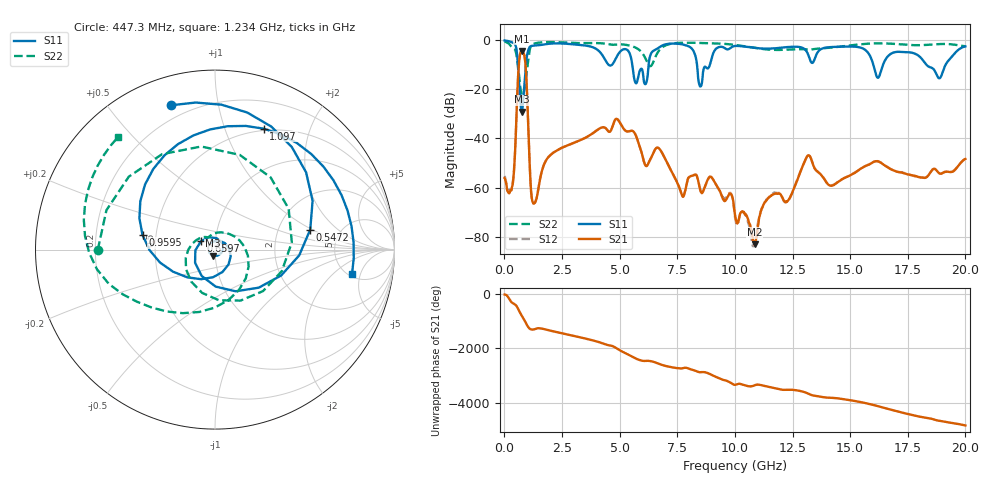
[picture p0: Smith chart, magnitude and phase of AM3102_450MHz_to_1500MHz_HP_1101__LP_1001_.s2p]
!Agilent Technologies,E8364B,MY43040894,A.07.50.67
!Agilent E8364B: A.07.50.67
!Date: Thursday, January 11, 2018 06:39:39
!Correction: S11(Full 2 Port(1,2))
!S21(Full 2 Port(1,2))
!S12(Full 2 Port(1,2))
!S22(Full 2 Port(1,2))
!S2P File: Measurements: S11, S21, S12, S22:
# Hz S  dB  R 50
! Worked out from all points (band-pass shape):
!   1601 points, 10 MHz to 20 GHz, reference 50 ohm
!   highest |S21| = -4.32 dB at 759.6 MHz (marker M1); lowest = -83.1 dB at 10.85 GHz (marker M2)
!   |S21| within 3 dB of the highest: 654.9 MHz to 886.7 MHz (231.9 MHz wide, 30.1 % of centre)
!   lowest |S11| = -29.0 dB at 747.1 MHz (marker M3), VSWR 1.07, Z = 48.8 - j3.27 ohm
!   |S11| at or under -10 dB: 5.549 GHz to 6.254 GHz (704.9 MHz wide, 11.9 % of centre); 8.358 GHz to 8.915 GHz (556.9 MHz wide, 6.45 % of centre); 18.31 GHz to 19.14 GHz (826.2 MHz wide, 4.41 % of centre)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
!   |S22| runs from -22.2 to -0.5 dB; largest |S21 - S12| = 0.0013
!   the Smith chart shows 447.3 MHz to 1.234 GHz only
!   S11 on the Smith chart (normalised r, x): 447.3 MHz: 0.13, +0.73; 547.2 MHz: 3.03, +0.96; 659.7 MHz: 0.85, +0.08; 959.5 MHz: 0.42, +0.08; 1.097 GHz: 0.48, +1.37; 1.234 GHz: 5.38, -3.64
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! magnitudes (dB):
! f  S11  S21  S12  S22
! 10 MHz  -0.1  -56.2  -55.3  -0.5
! 284.9 MHz  -0.7  -61.0  -60.4  -2.5
! 447.3 MHz  -1.5  -48.7  -48.1  -3.7
! 547.2 MHz  -5.3  -24.6  -24.6  -7.3
! 659.7 MHz  -20.8  -6.9  -6.9  -16.6
! 747.1 MHz  -29.0  -4.3  -4.3  -21.7
! 759.6 MHz  -29.0  -4.3  -4.3  -22.0
! 959.5 MHz  -7.7  -16.5  -16.5  -13.6
! 1.097 GHz  -2.8  -50.5  -50.7  -4.1
! 1.234 GHz  -2.2  -66.1  -66.2  -1.6
! 3.346 GHz  -2.0  -40.5  -40.5  -1.1
! 4.895 GHz  -6.4  -32.1  -32.1  -1.7
! 6.119 GHz  -17.9  -51.0  -51.0  -7.4
! 6.682 GHz  -3.1  -43.9  -43.9  -4.5
! 8.081 GHz  -3.0  -55.3  -55.4  -1.0
! 8.493 GHz  -18.8  -60.9  -60.8  -1.1
! 10.01 GHz  -2.3  -71.3  -72.1  -1.9
! 10.85 GHz  -3.1  -83.1  -82.8  -3.1
! 13.34 GHz  -9.2  -49.2  -49.1  -3.7
! 16.68 GHz  -6.1  -52.0  -52.0  -1.3
! 18.86 GHz  -15.5  -54.2  -54.2  -1.5
! 20 GHz  -2.5  -48.3  -48.2  -2.4
